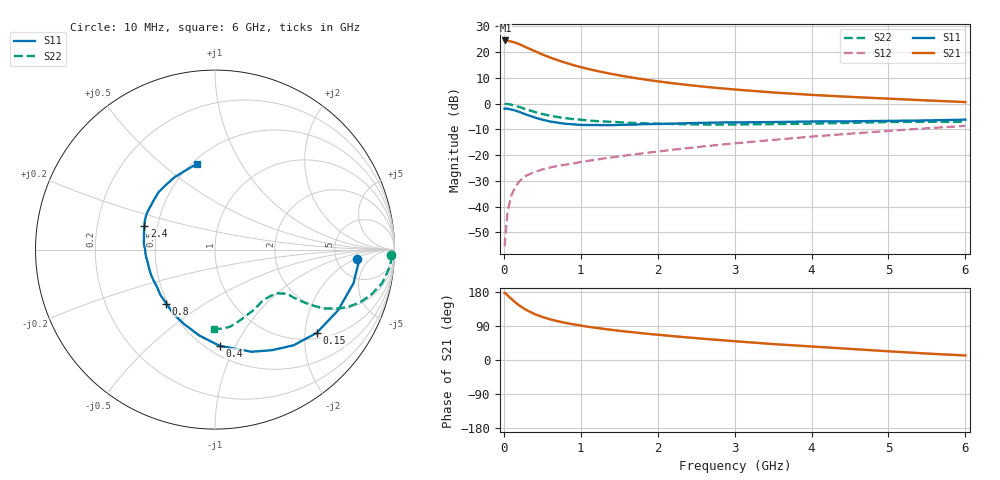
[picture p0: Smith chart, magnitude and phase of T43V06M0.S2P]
! Infineon Technologies  Discrete & RF Semiconductors
! BFR182T
! Si NPN RF Bipolar Junction Transistor in SC75
! VCE = 3 V  IC = 6 mA
! Common Emitter S-Parameters:  October  1999
# GHz  S  MA  R  50
!  f  S11  S21  S12  S22
! GHz  MAG  ANG  MAG  ANG  MAG  ANG  MAG  ANG
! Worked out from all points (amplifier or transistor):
!   36 points, 10 MHz to 6 GHz, reference 50 ohm
!   highest |S21| = 24.5 dB at 20 MHz (marker M1)
!   |S21| within 3 dB of that: start of sweep to 316.1 MHz
!   unconditionally stable (mu >= 1): 1.304 GHz to 3.952 GHz
!   at 250 MHz: K = 0.32, MSG = 25.6 dB, |S12| = -28.8 dB
!   at 1.4 GHz: K = 1.03, MAG = 15.2 dB, |S12| = -20.9 dB
!   at 6 GHz: K = 0.84, MSG = 4.6 dB, |S12| = -8.7 dB
!   lowest NFmin = 1.25 dB at 450 MHz
!   S11 on the Smith chart (normalised r, x): 10 MHz: 7.92, -2.28; 150 MHz: 1.15, -2.30; 400 MHz: 0.58, -0.87; 800 MHz: 0.49, -0.35; 2.4 GHz: 0.42, +0.14; 6 GHz: 0.53, +0.66
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0.01  0.7915 -3.9  16.72 177.1  0.0017 88.1  0.9824 -1.9
0.02  0.8053 -4.2  16.82 176.2  0.0026 91.5  0.9857 -2.4
0.05  0.7941 -13.7  16.63 170.1  0.0082 84.8  0.9776 -5.9
0.1  0.7641 -26.4  15.99 160.9  0.0169 79.1  0.95 -11.3
0.15  0.732 -39.4  15.22 151.9  0.0242 70.8  0.9065 -16.0
0.2  0.6898 -50.6  14.26 144.2  0.0306 67.8  0.8613 -19.9
0.25  0.6441 -60.5  13.2 137.3  0.0361 62.9  0.811 -23.0
0.3  0.6045 -70.3  12.21 131.2  0.0404 60.9  0.7673 -25.3
0.4  0.5371 -87.1  10.46 121.2  0.0468 56.5  0.6874 -28.5
0.5  0.4861 -100.6  9.008 113.7  0.0524 54.6  0.6286 -29.7
0.6  0.4485 -112.8  7.848 107.4  0.0572 54.1  0.5831 -30.6
0.7  0.4262 -123.1  6.95 102.4  0.0615 54.4  0.5475 -31.0
0.8  0.405 -132.1  6.222 98.0  0.065 53.8  0.5208 -31.3
1.1  0.3831 -153.9  4.694 87.5  0.0776 56.0  0.4699 -32.1
1.3  0.3817 -164.9  4.035 82.1  0.086 57.5  0.4483 -33.0
1.6  0.3887 -177.6  3.322 74.8  0.0988 59.4  0.4256 -34.8
2.2  0.4082 165.6  2.477 62.9  0.1271 62.1  0.4013 -40.8
2.4  0.4154 161.2  2.287 59.4  0.137 62.5  0.3947 -43.3
3.5  0.4374 141.8  1.644 42.0  0.197 62.1  0.3994 -57.6
4.5  0.4521 127.7  1.35 29.3  0.2602 59.0  0.4218 -72.1
5.5  0.4704 110.5  1.151 17.0  0.3313 54.1  0.4427 -85.1
6  0.4874 102.2  1.07 12.0  0.3692 50.7  0.442 -90.6
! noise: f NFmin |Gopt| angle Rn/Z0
0.45  1.25  0.25  39  0.3
0.9  1.4  0.25  78  0.23
1.8  1.95  0.21  151  0.2
